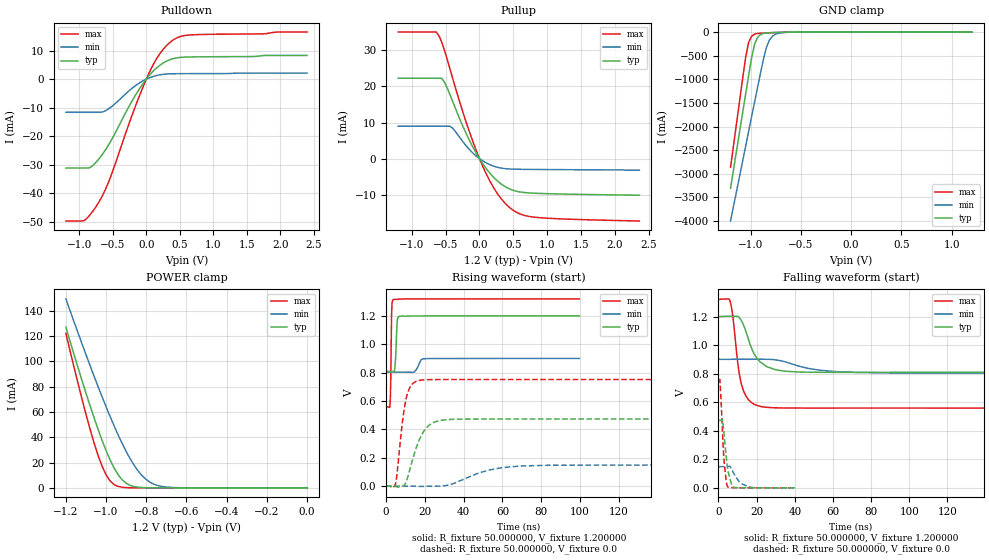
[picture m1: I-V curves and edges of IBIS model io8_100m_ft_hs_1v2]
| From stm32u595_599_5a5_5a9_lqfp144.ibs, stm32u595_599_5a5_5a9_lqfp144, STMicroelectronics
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|   Model io8_100m_ft_hs_1v2
[Model]  io8_100m_ft_hs_1v2
Model_type I/O
Polarity   Non-Inverting
Enable   Active-Low
Vinl =   0.360000V
Vinh =   0.840000V
Vmeas =  0.600000V
Cref =   50.000000pF
Rref =   100.000000M
Vref =   0.0V
C_comp   2.947800pF   2.877700pF   2.996100pF
[Temperature Range]   25.000000   0.140000k   -40.000000
[Pullup Reference]   1.200000V   0.900000V   1.320000V
[Pulldown Reference]   0.0V   0.0V   0.0V
[POWER Clamp Reference]   1.200000V   0.900000V   1.320000V
[GND Clamp Reference]   0.0V   0.0V   0.0V
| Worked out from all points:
|   slope of the pulldown table from 0 to 0.18 V, typ, clamps not added: 40.7 ohm
|   slope of the pullup table from 0 to 0.18 V, typ, clamps not added: 39.5 ohm
|   GND clamp passes 1 mA (typ) near -0.51 V on its own axis
|   POWER clamp passes 1 mA (typ) near -0.86 V on its own axis
|   rising waveform, R_fixture 50.000000, V_fixture 1.200000: 20-80 % time 753ps typ, 2.05ns min, 443ps max; typ from 0.809 V to 1.2 V
|   rising waveform, R_fixture 50.000000, V_fixture 0.0: 20-80 % time 7.25ns typ, 18.3ns min, 3.99ns max; typ from 0 V to 0.473 V
|   falling waveform, R_fixture 50.000000, V_fixture 1.200000: 20-80 % time 7.8ns typ, 18.5ns min, 4.53ns max; typ from 1.2 V to 0.809 V
|   falling waveform, R_fixture 50.000000, V_fixture 0.0: 20-80 % time 2.5ns typ, 4.76ns min, 1.85ns max; typ from 0.473 V to 0 V
[Pulldown]
|Voltage   I(typ)   I(min)   I(max)
-1.2V     -31.16mA   -11.61mA   -49.71mA
-920mV    -31.16mA   -11.61mA   -49.48mA
-840mV    -31mA      -11.61mA   -47.54mA
-720mV    -28.32mA   -11.61mA   -43.58mA
-560mV    -22.95mA   -10.37mA   -35.89mA
-200mV    -7.146mA   -2.964mA   -11.89mA
0V        0A         0A         0A
160mV     4.047mA    1.298mA    7.361mA
360mV     6.87mA     1.87mA     13mA
480mV     7.543mA    1.91mA     14.69mA
640mV     7.764mA    1.923mA    15.46mA
2.4V      8.308mA    2.101mA    16.5mA
[Pullup]
|Voltage   I(typ)   I(min)   I(max)
-1.2V     22.25mA    8.971mA    35.01mA
-640mV    22.25mA    8.971mA    35.01mA
-600mV    22.25mA    8.971mA    34.03mA
-520mV    21.23mA    8.971mA    30.12mA
-400mV    15.99mA    8.489mA    22.45mA
-200mV    7.069mA    3.642mA    10.26mA
0V        550fA      209pA      10fA
240mV     -5.73mA    -2.256mA   -8.953mA
480mV     -8.639mA   -2.877mA   -14.04mA
640mV     -9.31mA    -2.942mA   -15.55mA
880mV     -9.601mA   -2.986mA   -16.29mA
2.36V     -10.1mA    -3.2mA     -17.23mA
[GND_clamp]
|Voltage   I(typ)   I(min)   I(max)
-1.2V     -3.305A    -3.998A    -2.862A
-1.05V    -1.316A    -2.418A    -539.3mA
-1.02V    -921mA     -2.103A    -218.8mA
-990mV    -539.5mA   -1.788A    -87.43mA
-960mV    -252.1mA   -1.474A    -44.36mA
-930mV    -110.5mA   -1.16A     -30.32mA
-870mV    -28.03mA   -549.1mA   -21.09mA
-840mV    -18.43mA   -305.6mA   -18.27mA
-810mV    -13.9mA    -159.7mA   -15.73mA
-780mV    -11.23mA   -82.35mA   -13.37mA
-600mV    -2.976mA   -4.272mA   -3.058mA
1.2V      0A         14.74nA    0A
[POWER_clamp]
|Voltage   I(typ)   I(min)   I(max)
-1.2V     127mA      149.4mA    122.2mA
-1.12V    84.97mA    114mA      70.27mA
-1.06V    55.51mA    88.42mA    35.67mA
-1.02V    37.63mA    72.04mA    17.17mA
-1V       29.51mA    64.13mA    10.3mA
-960mV    15.69mA    48.99mA    2.571mA
-900mV    3.624mA    28.77mA    182.8uA
-840mV    490.7uA    13.24mA    11.35uA
-800mV    116.8uA    6.532mA    1.77uA
-740mV    13.2uA     1.723mA    109.1nA
-620mV    167.3nA    79.35uA    0A
0V        0A         17.84nA    0A
[Ramp]
| variable   typ   min   max
dV/dt_r  0.28375/7.23373n   88.91387m/18.29687n 0.45093/3.98286n
dV/dt_f  0.23460/7.78508n   57.88800m/18.44549n 0.45665/4.52035n
R_load = 50.000000
[Rising Waveform]
R_fixture= 50.000000
V_fixture= 1.200000
V_fixture_min= 0.900000
V_fixture_max= 1.320000
|time   V(typ)   V(min)   V(max)
0s        809mV      803.5mV    558.9mV
2.002ns   809mV      803.5mV    575mV
2.402ns   809.1mV    803.5mV    766.2mV
2.803ns   809mV      803.5mV    1.211V
3.804ns   804.9mV    803.5mV    1.315V
4.605ns   852.3mV    803.5mV    1.317V
5.806ns   1.173V     803.5mV    1.317V
6.807ns   1.196V     803.5mV    1.318V
19.62ns   1.2V       898.1mV    1.32V
99.7ns    1.2V       900mV      1.32V
[Rising Waveform]
R_fixture= 50.000000
V_fixture= 0.0
V_fixture_min= 0.0
V_fixture_max= 0.0
|time   V(typ)   V(min)   V(max)
0s        1.836uV    1.092uV    1.941uV
4.805ns   -2.478mV   913nV      12.66mV
8.408ns   -280.3uV   -122nV     453.8mV
10.21ns   26.56mV    1.793uV    609.6mV
12.61ns   136mV      48.02uV    704.5mV
16.82ns   318.1mV    -1.253mV   744.3mV
24.02ns   446.1mV    -17.07uV   751.1mV
34.23ns   470.8mV    16.32mV    751.4mV
69.07ns   472.8mV    141.6mV    751.5mV
299.1ns   472.9mV    148.2mV    751.5mV
[Falling Waveform]
R_fixture= 50.000000
V_fixture= 1.200000
V_fixture_min= 0.900000
V_fixture_max= 1.320000
|time   V(typ)   V(min)   V(max)
0s        1.2V       900mV      1.32V
6.006ns   1.201V     900.1mV    1.311V
7.608ns   1.202V     900.6mV    1.191V
10.81ns   1.194V     900.6mV    805mV
12.01ns   1.171V     900.5mV    726.7mV
15.62ns   1.044V     900.4mV    619.4mV
20.82ns   897.2mV    900.5mV    574.5mV
30.03ns   826.9mV    896mV      560.7mV
42.84ns   810.8mV    850mV      559mV
199.4ns   809mV      803.5mV    558.9mV
[Falling Waveform]
R_fixture= 50.000000
V_fixture= 0.0
V_fixture_min= 0.0
V_fixture_max= 0.0
|time   V(typ)   V(min)   V(max)
0s        472.9mV    148.2mV    751.5mV
800.8ps   472.9mV    148.3mV    743.2mV
2.162ns   473.5mV    148.3mV    371.2mV
3.043ns   357.3mV    148.2mV    172.6mV
4.645ns   150.1mV    148.4mV    10.08mV
6.567ns   36.23mV    138mV      2.166mV
7.928ns   3.374mV    103.5mV    1.055mV
11.61ns   1.113mV    34mV       295.9uV
17.38ns   296.1uV    2.863mV    67.7uV
39.88ns   1.836uV    1.092uV    1.941uV
